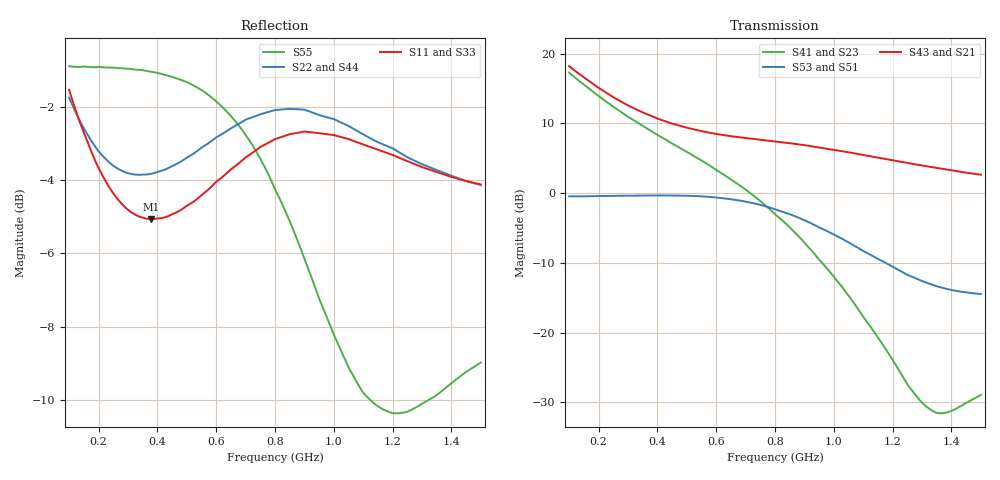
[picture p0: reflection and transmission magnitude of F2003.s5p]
!  POLYFET RF DEVICES
!  S PARAMETERS FOR
!  F2003 (Each Side)
!  VDS=28, IDQ=200mA
! Date: Mon Aug  5 14:30:38 1991
!AWR Design Environment (2053) Thu Feb 05 14:06:27 2004
!freq-unit  param-type  data-format  keyword  impedance-ohms
# MHz  S  MA  R  50
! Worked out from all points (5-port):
!   141 points, 100 MHz to 1.5 GHz, reference 50 ohm
!   strongest paths, dB at 100 MHz, 450 MHz, 800 MHz, 1.15 GHz, 1.5 GHz:
!     S43: 18.2, 10.0, 7.4, 5.1, 2.6
!     S21: 18.2, 10.0, 7.4, 5.1, 2.6
!     S53: -0.5, -0.4, -2.3, -9.4, -14.5
!     S51: -0.5, -0.4, -2.3, -9.4, -14.5
!     S41: 17.3, 7.1, -3.0, -20.7, -29.0
!     S23: 17.3, 7.1, -3.0, -20.7, -29.0
!   lowest |S11| = -5.1 dB at 380 MHz (marker M1), VSWR 3.52, Z = 39.9 - j59.1 ohm
!   |S11| at or under -10 dB: nowhere
